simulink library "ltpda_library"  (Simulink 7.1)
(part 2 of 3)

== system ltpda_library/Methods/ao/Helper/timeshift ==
  In1 : Inport  OutDataType=sfix(16)  OutScaling=2^0
  timeshift : M-S-Function  Tag=timeshift  FunctionName=ltpdasim
  Out1 : Outport  OutDataType=sfix(16)  OutScaling=2^0
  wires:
  In1/1 -> timeshift/1
  timeshift/1 -> Out1/1

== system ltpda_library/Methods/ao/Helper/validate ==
  In1 : Inport  OutDataType=sfix(16)  OutScaling=2^0
  validate : M-S-Function  Tag=validate  FunctionName=ltpdasim
  Out1 : Outport  OutDataType=sfix(16)  OutScaling=2^0
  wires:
  In1/1 -> validate/1
  validate/1 -> Out1/1

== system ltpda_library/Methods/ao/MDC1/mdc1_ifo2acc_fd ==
  In1 : Inport  OutDataType=sfix(16)  OutScaling=2^0
  mdc1_ifo2acc_fd : M-S-Function  Tag=mdc1_ifo2acc_fd  FunctionName=ltpdasim
  Out1 : Outport  OutDataType=sfix(16)  OutScaling=2^0
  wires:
  In1/1 -> mdc1_ifo2acc_fd/1
  mdc1_ifo2acc_fd/1 -> Out1/1

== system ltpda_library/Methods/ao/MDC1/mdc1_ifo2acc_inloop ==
  In1 : Inport  OutDataType=sfix(16)  OutScaling=2^0
  mdc1_ifo2acc_inloop : M-S-Function  Tag=mdc1_ifo2acc_inloop  FunctionName=ltpdasim
  Out1 : Outport  OutDataType=sfix(16)  OutScaling=2^0
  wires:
  In1/1 -> mdc1_ifo2acc_inloop/1
  mdc1_ifo2acc_inloop/1 -> Out1/1

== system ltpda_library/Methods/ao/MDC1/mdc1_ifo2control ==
  In1 : Inport  OutDataType=sfix(16)  OutScaling=2^0
  mdc1_ifo2control : M-S-Function  Tag=mdc1_ifo2control  FunctionName=ltpdasim
  Out1 : Outport  OutDataType=sfix(16)  OutScaling=2^0
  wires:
  In1/1 -> mdc1_ifo2control/1
  mdc1_ifo2control/1 -> Out1/1

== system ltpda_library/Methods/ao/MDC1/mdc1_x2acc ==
  In1 : Inport  OutDataType=sfix(16)  OutScaling=2^0
  mdc1_x2acc : M-S-Function  Tag=mdc1_x2acc  FunctionName=ltpdasim
  Out1 : Outport  OutDataType=sfix(16)  OutScaling=2^0
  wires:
  In1/1 -> mdc1_x2acc/1
  mdc1_x2acc/1 -> Out1/1

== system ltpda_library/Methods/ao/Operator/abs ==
  In1 : Inport  OutDataType=sfix(16)  OutScaling=2^0
  abs : M-S-Function  Tag=abs  FunctionName=ltpdasim
  Out1 : Outport  OutDataType=sfix(16)  OutScaling=2^0
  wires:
  In1/1 -> abs/1
  abs/1 -> Out1/1

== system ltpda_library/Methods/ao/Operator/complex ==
  In1 : Inport  OutDataType=sfix(16)  OutScaling=2^0
  complex : M-S-Function  Tag=complex  FunctionName=ltpdasim
  Out1 : Outport  OutDataType=sfix(16)  OutScaling=2^0
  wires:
  In1/1 -> complex/1
  complex/1 -> Out1/1

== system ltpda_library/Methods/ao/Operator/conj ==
  In1 : Inport  OutDataType=sfix(16)  OutScaling=2^0
  conj : M-S-Function  Tag=conj  FunctionName=ltpdasim
  Out1 : Outport  OutDataType=sfix(16)  OutScaling=2^0
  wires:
  In1/1 -> conj/1
  conj/1 -> Out1/1

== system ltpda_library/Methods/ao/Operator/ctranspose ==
  In1 : Inport  OutDataType=sfix(16)  OutScaling=2^0
  ctranspose : M-S-Function  Tag=ctranspose  FunctionName=ltpdasim
  Out1 : Outport  OutDataType=sfix(16)  OutScaling=2^0
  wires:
  In1/1 -> ctranspose/1
  ctranspose/1 -> Out1/1

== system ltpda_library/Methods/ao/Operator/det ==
  In1 : Inport  OutDataType=sfix(16)  OutScaling=2^0
  det : M-S-Function  Tag=det  FunctionName=ltpdasim
  Out1 : Outport  OutDataType=sfix(16)  OutScaling=2^0
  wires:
  In1/1 -> det/1
  det/1 -> Out1/1

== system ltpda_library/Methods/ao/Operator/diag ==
  In1 : Inport  OutDataType=sfix(16)  OutScaling=2^0
  diag : M-S-Function  Tag=diag  FunctionName=ltpdasim
  Out1 : Outport  OutDataType=sfix(16)  OutScaling=2^0
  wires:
  In1/1 -> diag/1
  diag/1 -> Out1/1

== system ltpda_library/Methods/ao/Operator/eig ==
  In1 : Inport  OutDataType=sfix(16)  OutScaling=2^0
  eig : M-S-Function  Tag=eig  FunctionName=ltpdasim
  Out1 : Outport  OutDataType=sfix(16)  OutScaling=2^0
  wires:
  In1/1 -> eig/1
  eig/1 -> Out1/1

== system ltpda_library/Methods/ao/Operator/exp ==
  In1 : Inport  OutDataType=sfix(16)  OutScaling=2^0
  exp : M-S-Function  Tag=exp  FunctionName=ltpdasim
  Out1 : Outport  OutDataType=sfix(16)  OutScaling=2^0
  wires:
  In1/1 -> exp/1
  exp/1 -> Out1/1

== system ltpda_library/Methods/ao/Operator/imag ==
  In1 : Inport  OutDataType=sfix(16)  OutScaling=2^0
  imag : M-S-Function  Tag=imag  FunctionName=ltpdasim
  Out1 : Outport  OutDataType=sfix(16)  OutScaling=2^0
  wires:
  In1/1 -> imag/1
  imag/1 -> Out1/1

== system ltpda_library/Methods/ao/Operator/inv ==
  In1 : Inport  OutDataType=sfix(16)  OutScaling=2^0
  inv : M-S-Function  Tag=inv  FunctionName=ltpdasim
  Out1 : Outport  OutDataType=sfix(16)  OutScaling=2^0
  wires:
  In1/1 -> inv/1
  inv/1 -> Out1/1

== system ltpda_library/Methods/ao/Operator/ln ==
  In1 : Inport  OutDataType=sfix(16)  OutScaling=2^0
  ln : M-S-Function  Tag=ln  FunctionName=ltpdasim
  Out1 : Outport  OutDataType=sfix(16)  OutScaling=2^0
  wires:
  In1/1 -> ln/1
  ln/1 -> Out1/1

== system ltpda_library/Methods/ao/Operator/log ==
  In1 : Inport  OutDataType=sfix(16)  OutScaling=2^0
  log : M-S-Function  Tag=log  FunctionName=ltpdasim
  Out1 : Outport  OutDataType=sfix(16)  OutScaling=2^0
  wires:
  In1/1 -> log/1
  log/1 -> Out1/1

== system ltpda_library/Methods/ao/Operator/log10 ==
  In1 : Inport  OutDataType=sfix(16)  OutScaling=2^0
  log10 : M-S-Function  Tag=log10  FunctionName=ltpdasim
  Out1 : Outport  OutDataType=sfix(16)  OutScaling=2^0
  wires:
  In1/1 -> log10/1
  log10/1 -> Out1/1

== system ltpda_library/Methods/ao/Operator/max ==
  In1 : Inport  OutDataType=sfix(16)  OutScaling=2^0
  max : M-S-Function  Tag=max  FunctionName=ltpdasim
  Out1 : Outport  OutDataType=sfix(16)  OutScaling=2^0
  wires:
  In1/1 -> max/1
  max/1 -> Out1/1

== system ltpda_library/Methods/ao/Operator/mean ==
  In1 : Inport  OutDataType=sfix(16)  OutScaling=2^0
  mean : M-S-Function  Tag=mean  FunctionName=ltpdasim
  Out1 : Outport  OutDataType=sfix(16)  OutScaling=2^0
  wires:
  In1/1 -> mean/1
  mean/1 -> Out1/1

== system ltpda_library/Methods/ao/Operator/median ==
  In1 : Inport  OutDataType=sfix(16)  OutScaling=2^0
  median : M-S-Function  Tag=median  FunctionName=ltpdasim
  Out1 : Outport  OutDataType=sfix(16)  OutScaling=2^0
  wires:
  In1/1 -> median/1
  median/1 -> Out1/1

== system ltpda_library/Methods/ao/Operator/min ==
  In1 : Inport  OutDataType=sfix(16)  OutScaling=2^0
  min : M-S-Function  Tag=min  FunctionName=ltpdasim
  Out1 : Outport  OutDataType=sfix(16)  OutScaling=2^0
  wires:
  In1/1 -> min/1
  min/1 -> Out1/1

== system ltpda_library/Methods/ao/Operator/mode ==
  In1 : Inport  OutDataType=sfix(16)  OutScaling=2^0
  mode : M-S-Function  Tag=mode  FunctionName=ltpdasim
  Out1 : Outport  OutDataType=sfix(16)  OutScaling=2^0
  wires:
  In1/1 -> mode/1
  mode/1 -> Out1/1

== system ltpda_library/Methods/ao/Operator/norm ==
  In1 : Inport  OutDataType=sfix(16)  OutScaling=2^0
  norm : M-S-Function  Tag=norm  FunctionName=ltpdasim
  Out1 : Outport  OutDataType=sfix(16)  OutScaling=2^0
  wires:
  In1/1 -> norm/1
  norm/1 -> Out1/1

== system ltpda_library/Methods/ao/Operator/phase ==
  In1 : Inport  OutDataType=sfix(16)  OutScaling=2^0
  phase : M-S-Function  Tag=phase  FunctionName=ltpdasim
  Out1 : Outport  OutDataType=sfix(16)  OutScaling=2^0
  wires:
  In1/1 -> phase/1
  phase/1 -> Out1/1

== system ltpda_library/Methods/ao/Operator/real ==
  In1 : Inport  OutDataType=sfix(16)  OutScaling=2^0
  real : M-S-Function  Tag=real  FunctionName=ltpdasim
  Out1 : Outport  OutDataType=sfix(16)  OutScaling=2^0
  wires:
  In1/1 -> real/1
  real/1 -> Out1/1

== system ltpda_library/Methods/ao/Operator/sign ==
  In1 : Inport  OutDataType=sfix(16)  OutScaling=2^0
  sign : M-S-Function  Tag=sign  FunctionName=ltpdasim
  Out1 : Outport  OutDataType=sfix(16)  OutScaling=2^0
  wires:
  In1/1 -> sign/1
  sign/1 -> Out1/1

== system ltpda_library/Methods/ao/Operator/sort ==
  In1 : Inport  OutDataType=sfix(16)  OutScaling=2^0
  sort : M-S-Function  Tag=sort  FunctionName=ltpdasim
  Out1 : Outport  OutDataType=sfix(16)  OutScaling=2^0
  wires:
  In1/1 -> sort/1
  sort/1 -> Out1/1

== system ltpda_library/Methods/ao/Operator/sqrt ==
  In1 : Inport  OutDataType=sfix(16)  OutScaling=2^0
  sqrt : M-S-Function  Tag=sqrt  FunctionName=ltpdasim
  Out1 : Outport  OutDataType=sfix(16)  OutScaling=2^0
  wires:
  In1/1 -> sqrt/1
  sqrt/1 -> Out1/1

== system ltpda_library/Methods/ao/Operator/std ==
  In1 : Inport  OutDataType=sfix(16)  OutScaling=2^0
  std : M-S-Function  Tag=std  FunctionName=ltpdasim
  Out1 : Outport  OutDataType=sfix(16)  OutScaling=2^0
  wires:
  In1/1 -> std/1
  std/1 -> Out1/1

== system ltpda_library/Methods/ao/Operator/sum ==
  In1 : Inport  OutDataType=sfix(16)  OutScaling=2^0
  sum : M-S-Function  Tag=sum  FunctionName=ltpdasim
  Out1 : Outport  OutDataType=sfix(16)  OutScaling=2^0
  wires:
  In1/1 -> sum/1
  sum/1 -> Out1/1

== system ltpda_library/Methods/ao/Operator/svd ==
  In1 : Inport  OutDataType=sfix(16)  OutScaling=2^0
  svd : M-S-Function  Tag=svd  FunctionName=ltpdasim
  Out1 : Outport  OutDataType=sfix(16)  OutScaling=2^0
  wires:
  In1/1 -> svd/1
  svd/1 -> Out1/1

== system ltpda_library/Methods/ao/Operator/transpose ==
  In1 : Inport  OutDataType=sfix(16)  OutScaling=2^0
  transpose : M-S-Function  Tag=transpose  FunctionName=ltpdasim
  Out1 : Outport  OutDataType=sfix(16)  OutScaling=2^0
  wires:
  In1/1 -> transpose/1
  transpose/1 -> Out1/1

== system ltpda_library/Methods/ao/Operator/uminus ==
  In1 : Inport  OutDataType=sfix(16)  OutScaling=2^0
  uminus : M-S-Function  Tag=uminus  FunctionName=ltpdasim
  Out1 : Outport  OutDataType=sfix(16)  OutScaling=2^0
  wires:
  In1/1 -> uminus/1
  uminus/1 -> Out1/1

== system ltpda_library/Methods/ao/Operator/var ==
  In1 : Inport  OutDataType=sfix(16)  OutScaling=2^0
  var : M-S-Function  Tag=var  FunctionName=ltpdasim
  Out1 : Outport  OutDataType=sfix(16)  OutScaling=2^0
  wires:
  In1/1 -> var/1
  var/1 -> Out1/1

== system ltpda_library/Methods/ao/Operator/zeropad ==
  In1 : Inport  OutDataType=sfix(16)  OutScaling=2^0
  zeropad : M-S-Function  Tag=zeropad  FunctionName=ltpdasim
  Out1 : Outport  OutDataType=sfix(16)  OutScaling=2^0
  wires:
  In1/1 -> zeropad/1
  zeropad/1 -> Out1/1

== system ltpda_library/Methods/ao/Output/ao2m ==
  In1 : Inport  OutDataType=sfix(16)  OutScaling=2^0
  Terminator : Terminator
  ao2m : M-S-Function  Tag=ao2m  FunctionName=ltpdasim
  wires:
  ao2m/1 -> Terminator/1
  In1/1 -> ao2m/1

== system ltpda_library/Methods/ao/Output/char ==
  In1 : Inport  OutDataType=sfix(16)  OutScaling=2^0
  Terminator : Terminator
  char : M-S-Function  Tag=char  FunctionName=ltpdasim
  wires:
  char/1 -> Terminator/1
  In1/1 -> char/1

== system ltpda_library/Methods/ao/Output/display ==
  In1 : Inport  OutDataType=sfix(16)  OutScaling=2^0
  Terminator : Terminator
  display : M-S-Function  Tag=display  FunctionName=ltpdasim
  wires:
  display/1 -> Terminator/1
  In1/1 -> display/1

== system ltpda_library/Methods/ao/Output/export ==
  In1 : Inport  OutDataType=sfix(16)  OutScaling=2^0
  Terminator : Terminator
  export : M-S-Function  Tag=export  FunctionName=ltpdasim
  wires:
  export/1 -> Terminator/1
  In1/1 -> export/1

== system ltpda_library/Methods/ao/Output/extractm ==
  In1 : Inport  OutDataType=sfix(16)  OutScaling=2^0
  Terminator : Terminator
  extractm : M-S-Function  Tag=extractm  FunctionName=ltpdasim
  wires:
  extractm/1 -> Terminator/1
  In1/1 -> extractm/1

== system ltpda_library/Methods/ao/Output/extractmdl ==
  In1 : Inport  OutDataType=sfix(16)  OutScaling=2^0
  Terminator : Terminator
  extractmdl : M-S-Function  Tag=extractmdl  FunctionName=ltpdasim
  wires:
  extractmdl/1 -> Terminator/1
  In1/1 -> extractmdl/1

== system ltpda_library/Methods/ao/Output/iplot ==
  In1 : Inport  OutDataType=sfix(16)  OutScaling=2^0
  Terminator : Terminator
  iplot : M-S-Function  Tag=iplot  FunctionName=ltpdasim
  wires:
  iplot/1 -> Terminator/1
  In1/1 -> iplot/1

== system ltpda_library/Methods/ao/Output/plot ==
  In1 : Inport  OutDataType=sfix(16)  OutScaling=2^0
  Terminator : Terminator
  plot : M-S-Function  Tag=plot  FunctionName=ltpdasim
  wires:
  plot/1 -> Terminator/1
  In1/1 -> plot/1

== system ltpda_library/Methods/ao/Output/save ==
  In1 : Inport  OutDataType=sfix(16)  OutScaling=2^0
  Terminator : Terminator
  save : M-S-Function  Tag=save  FunctionName=ltpdasim
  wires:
  save/1 -> Terminator/1
  In1/1 -> save/1

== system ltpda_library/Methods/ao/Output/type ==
  In1 : Inport  OutDataType=sfix(16)  OutScaling=2^0
  Terminator : Terminator
  type : M-S-Function  Tag=type  FunctionName=ltpdasim
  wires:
  type/1 -> Terminator/1
  In1/1 -> type/1

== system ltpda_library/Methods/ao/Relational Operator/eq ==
  In1 : Inport  OutDataType=sfix(16)  OutScaling=2^0
  eq : M-S-Function  Tag=eq  FunctionName=ltpdasim
  Out1 : Outport  OutDataType=sfix(16)  OutScaling=2^0
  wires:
  In1/1 -> eq/1
  eq/1 -> Out1/1

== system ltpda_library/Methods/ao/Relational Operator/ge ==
  In1 : Inport  OutDataType=sfix(16)  OutScaling=2^0
  ge : M-S-Function  Tag=ge  FunctionName=ltpdasim
  Out1 : Outport  OutDataType=sfix(16)  OutScaling=2^0
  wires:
  In1/1 -> ge/1
  ge/1 -> Out1/1

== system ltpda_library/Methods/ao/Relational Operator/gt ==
  In1 : Inport  OutDataType=sfix(16)  OutScaling=2^0
  gt : M-S-Function  Tag=gt  FunctionName=ltpdasim
  Out1 : Outport  OutDataType=sfix(16)  OutScaling=2^0
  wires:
  In1/1 -> gt/1
  gt/1 -> Out1/1

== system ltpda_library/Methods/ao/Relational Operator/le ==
  In1 : Inport  OutDataType=sfix(16)  OutScaling=2^0
  le : M-S-Function  Tag=le  FunctionName=ltpdasim
  Out1 : Outport  OutDataType=sfix(16)  OutScaling=2^0
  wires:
  In1/1 -> le/1
  le/1 -> Out1/1

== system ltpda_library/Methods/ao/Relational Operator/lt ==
  In1 : Inport  OutDataType=sfix(16)  OutScaling=2^0
  lt : M-S-Function  Tag=lt  FunctionName=ltpdasim
  Out1 : Outport  OutDataType=sfix(16)  OutScaling=2^0
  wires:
  In1/1 -> lt/1
  lt/1 -> Out1/1

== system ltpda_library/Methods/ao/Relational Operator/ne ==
  In1 : Inport  OutDataType=sfix(16)  OutScaling=2^0
  ne : M-S-Function  Tag=ne  FunctionName=ltpdasim
  Out1 : Outport  OutDataType=sfix(16)  OutScaling=2^0
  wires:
  In1/1 -> ne/1
  ne/1 -> Out1/1

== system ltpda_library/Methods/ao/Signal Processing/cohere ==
  In1 : Inport  OutDataType=sfix(16)  OutScaling=2^0
  cohere : M-S-Function  Tag=cohere  FunctionName=ltpdasim
  Out1 : Outport  OutDataType=sfix(16)  OutScaling=2^0
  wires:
  In1/1 -> cohere/1
  cohere/1 -> Out1/1

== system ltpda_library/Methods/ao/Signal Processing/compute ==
  In1 : Inport  OutDataType=sfix(16)  OutScaling=2^0
  compute : M-S-Function  Tag=compute  FunctionName=ltpdasim
  Out1 : Outport  OutDataType=sfix(16)  OutScaling=2^0
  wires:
  In1/1 -> compute/1
  compute/1 -> Out1/1

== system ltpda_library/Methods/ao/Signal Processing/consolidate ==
  In1 : Inport  OutDataType=sfix(16)  OutScaling=2^0
  consolidate : M-S-Function  Tag=consolidate  FunctionName=ltpdasim
  Out1 : Outport  OutDataType=sfix(16)  OutScaling=2^0
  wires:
  In1/1 -> consolidate/1
  consolidate/1 -> Out1/1

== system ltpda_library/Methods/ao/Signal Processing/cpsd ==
  In1 : Inport  OutDataType=sfix(16)  OutScaling=2^0
  cpsd : M-S-Function  Tag=cpsd  FunctionName=ltpdasim
  Out1 : Outport  OutDataType=sfix(16)  OutScaling=2^0
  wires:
  In1/1 -> cpsd/1
  cpsd/1 -> Out1/1

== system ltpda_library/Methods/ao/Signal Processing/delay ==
  In1 : Inport  OutDataType=sfix(16)  OutScaling=2^0
  delay : M-S-Function  Tag=delay  FunctionName=ltpdasim
  Out1 : Outport  OutDataType=sfix(16)  OutScaling=2^0
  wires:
  In1/1 -> delay/1
  delay/1 -> Out1/1

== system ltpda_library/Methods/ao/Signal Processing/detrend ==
  In1 : Inport  OutDataType=sfix(16)  OutScaling=2^0
  detrend : M-S-Function  Tag=detrend  FunctionName=ltpdasim
  Out1 : Outport  OutDataType=sfix(16)  OutScaling=2^0
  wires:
  In1/1 -> detrend/1
  detrend/1 -> Out1/1

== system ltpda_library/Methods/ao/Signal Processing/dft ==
  In1 : Inport  OutDataType=sfix(16)  OutScaling=2^0
  dft : M-S-Function  Tag=dft  FunctionName=ltpdasim
  Out1 : Outport  OutDataType=sfix(16)  OutScaling=2^0
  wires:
  In1/1 -> dft/1
  dft/1 -> Out1/1

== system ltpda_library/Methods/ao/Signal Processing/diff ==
  In1 : Inport  OutDataType=sfix(16)  OutScaling=2^0
  diff : M-S-Function  Tag=diff  FunctionName=ltpdasim
  Out1 : Outport  OutDataType=sfix(16)  OutScaling=2^0
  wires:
  In1/1 -> diff/1
  diff/1 -> Out1/1

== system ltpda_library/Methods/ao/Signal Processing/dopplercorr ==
  In1 : Inport  OutDataType=sfix(16)  OutScaling=2^0
  dopplercorr : M-S-Function  Tag=dopplercorr  FunctionName=ltpdasim
  Out1 : Outport  OutDataType=sfix(16)  OutScaling=2^0
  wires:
  In1/1 -> dopplercorr/1
  dopplercorr/1 -> Out1/1

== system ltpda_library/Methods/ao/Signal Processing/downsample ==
  In1 : Inport  OutDataType=sfix(16)  OutScaling=2^0
  downsample : M-S-Function  Tag=downsample  FunctionName=ltpdasim
  Out1 : Outport  OutDataType=sfix(16)  OutScaling=2^0
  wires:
  In1/1 -> downsample/1
  downsample/1 -> Out1/1

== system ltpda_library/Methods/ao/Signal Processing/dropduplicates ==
  In1 : Inport  OutDataType=sfix(16)  OutScaling=2^0
  dropduplicates : M-S-Function  Tag=dropduplicates  FunctionName=ltpdasim
  Out1 : Outport  OutDataType=sfix(16)  OutScaling=2^0
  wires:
  In1/1 -> dropduplicates/1
  dropduplicates/1 -> Out1/1

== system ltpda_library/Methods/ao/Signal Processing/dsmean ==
  In1 : Inport  OutDataType=sfix(16)  OutScaling=2^0
  dsmean : M-S-Function  Tag=dsmean  FunctionName=ltpdasim
  Out1 : Outport  OutDataType=sfix(16)  OutScaling=2^0
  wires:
  In1/1 -> dsmean/1
  dsmean/1 -> Out1/1

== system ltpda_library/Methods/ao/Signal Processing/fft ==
  In1 : Inport  OutDataType=sfix(16)  OutScaling=2^0
  fft : M-S-Function  Tag=fft  FunctionName=ltpdasim
  Out1 : Outport  OutDataType=sfix(16)  OutScaling=2^0
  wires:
  In1/1 -> fft/1
  fft/1 -> Out1/1

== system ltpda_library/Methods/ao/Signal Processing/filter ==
  In1 : Inport  OutDataType=sfix(16)  OutScaling=2^0
  filter : M-S-Function  Tag=filter  FunctionName=ltpdasim
  Out1 : Outport  OutDataType=sfix(16)  OutScaling=2^0
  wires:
  In1/1 -> filter/1
  filter/1 -> Out1/1

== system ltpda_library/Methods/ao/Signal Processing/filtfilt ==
  In1 : Inport  OutDataType=sfix(16)  OutScaling=2^0
  filtfilt : M-S-Function  Tag=filtfilt  FunctionName=ltpdasim
  Out1 : Outport  OutDataType=sfix(16)  OutScaling=2^0
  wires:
  In1/1 -> filtfilt/1
  filtfilt/1 -> Out1/1

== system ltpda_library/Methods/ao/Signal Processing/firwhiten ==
  In1 : Inport  OutDataType=sfix(16)  OutScaling=2^0
  firwhiten : M-S-Function  Tag=firwhiten  FunctionName=ltpdasim
  Out1 : Outport  OutDataType=sfix(16)  OutScaling=2^0
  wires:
  In1/1 -> firwhiten/1
  firwhiten/1 -> Out1/1

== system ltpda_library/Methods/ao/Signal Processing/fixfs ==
  In1 : Inport  OutDataType=sfix(16)  OutScaling=2^0
  fixfs : M-S-Function  Tag=fixfs  FunctionName=ltpdasim
  Out1 : Outport  OutDataType=sfix(16)  OutScaling=2^0
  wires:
  In1/1 -> fixfs/1
  fixfs/1 -> Out1/1

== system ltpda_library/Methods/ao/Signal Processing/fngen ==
  In1 : Inport  OutDataType=sfix(16)  OutScaling=2^0
  fngen : M-S-Function  Tag=fngen  FunctionName=ltpdasim
  Out1 : Outport  OutDataType=sfix(16)  OutScaling=2^0
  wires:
  In1/1 -> fngen/1
  fngen/1 -> Out1/1

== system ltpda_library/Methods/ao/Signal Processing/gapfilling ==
  In1 : Inport  OutDataType=sfix(16)  OutScaling=2^0
  gapfilling : M-S-Function  Tag=gapfilling  FunctionName=ltpdasim
  Out1 : Outport  OutDataType=sfix(16)  OutScaling=2^0
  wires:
  In1/1 -> gapfilling/1
  gapfilling/1 -> Out1/1

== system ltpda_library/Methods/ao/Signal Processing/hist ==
  In1 : Inport  OutDataType=sfix(16)  OutScaling=2^0
  hist : M-S-Function  Tag=hist  FunctionName=ltpdasim
  Out1 : Outport  OutDataType=sfix(16)  OutScaling=2^0
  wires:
  In1/1 -> hist/1
  hist/1 -> Out1/1

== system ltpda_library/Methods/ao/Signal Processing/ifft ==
  In1 : Inport  OutDataType=sfix(16)  OutScaling=2^0
  ifft : M-S-Function  Tag=ifft  FunctionName=ltpdasim
  Out1 : Outport  OutDataType=sfix(16)  OutScaling=2^0
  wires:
  In1/1 -> ifft/1
  ifft/1 -> Out1/1

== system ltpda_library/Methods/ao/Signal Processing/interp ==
  In1 : Inport  OutDataType=sfix(16)  OutScaling=2^0
  interp : M-S-Function  Tag=interp  FunctionName=ltpdasim
  Out1 : Outport  OutDataType=sfix(16)  OutScaling=2^0
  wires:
  In1/1 -> interp/1
  interp/1 -> Out1/1

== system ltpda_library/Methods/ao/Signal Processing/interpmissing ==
  In1 : Inport  OutDataType=sfix(16)  OutScaling=2^0
  interpmissing : M-S-Function  Tag=interpmissing  FunctionName=ltpdasim
  Out1 : Outport  OutDataType=sfix(16)  OutScaling=2^0
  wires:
  In1/1 -> interpmissing/1
  interpmissing/1 -> Out1/1

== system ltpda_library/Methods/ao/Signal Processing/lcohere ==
  In1 : Inport  OutDataType=sfix(16)  OutScaling=2^0
  lcohere : M-S-Function  Tag=lcohere  FunctionName=ltpdasim
  Out1 : Outport  OutDataType=sfix(16)  OutScaling=2^0
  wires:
  In1/1 -> lcohere/1
  lcohere/1 -> Out1/1

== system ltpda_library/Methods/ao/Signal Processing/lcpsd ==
  In1 : Inport  OutDataType=sfix(16)  OutScaling=2^0
  lcpsd : M-S-Function  Tag=lcpsd  FunctionName=ltpdasim
  Out1 : Outport  OutDataType=sfix(16)  OutScaling=2^0
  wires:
  In1/1 -> lcpsd/1
  lcpsd/1 -> Out1/1

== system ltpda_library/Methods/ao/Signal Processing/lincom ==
  In1 : Inport  OutDataType=sfix(16)  OutScaling=2^0
  lincom : M-S-Function  Tag=lincom  FunctionName=ltpdasim
  Out1 : Outport  OutDataType=sfix(16)  OutScaling=2^0
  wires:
  In1/1 -> lincom/1
  lincom/1 -> Out1/1

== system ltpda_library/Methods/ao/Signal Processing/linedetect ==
  In1 : Inport  OutDataType=sfix(16)  OutScaling=2^0
  linedetect : M-S-Function  Tag=linedetect  FunctionName=ltpdasim
  Out1 : Outport  OutDataType=sfix(16)  OutScaling=2^0
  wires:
  In1/1 -> linedetect/1
  linedetect/1 -> Out1/1

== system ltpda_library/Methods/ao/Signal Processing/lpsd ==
  In1 : Inport  OutDataType=sfix(16)  OutScaling=2^0
  lpsd : M-S-Function  Tag=lpsd  FunctionName=ltpdasim
  Out1 : Outport  OutDataType=sfix(16)  OutScaling=2^0
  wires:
  In1/1 -> lpsd/1
  lpsd/1 -> Out1/1

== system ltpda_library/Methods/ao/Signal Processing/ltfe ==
  In1 : Inport  OutDataType=sfix(16)  OutScaling=2^0
  ltfe : M-S-Function  Tag=ltfe  FunctionName=ltpdasim
  Out1 : Outport  OutDataType=sfix(16)  OutScaling=2^0
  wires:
  In1/1 -> ltfe/1
  ltfe/1 -> Out1/1

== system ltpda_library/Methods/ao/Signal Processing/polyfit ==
  In1 : Inport  OutDataType=sfix(16)  OutScaling=2^0
  polyfit : M-S-Function  Tag=polyfit  FunctionName=ltpdasim
  Out1 : Outport  OutDataType=sfix(16)  OutScaling=2^0
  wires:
  In1/1 -> polyfit/1
  polyfit/1 -> Out1/1

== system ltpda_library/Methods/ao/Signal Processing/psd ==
  In1 : Inport  OutDataType=sfix(16)  OutScaling=2^0
  psd : M-S-Function  Tag=psd  FunctionName=ltpdasim
  Out1 : Outport  OutDataType=sfix(16)  OutScaling=2^0
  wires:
  In1/1 -> psd/1
  psd/1 -> Out1/1

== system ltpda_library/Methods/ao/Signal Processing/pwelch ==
  In1 : Inport  OutDataType=sfix(16)  OutScaling=2^0
  pwelch : M-S-Function  Tag=pwelch  FunctionName=ltpdasim
  Out1 : Outport  OutDataType=sfix(16)  OutScaling=2^0
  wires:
  In1/1 -> pwelch/1
  pwelch/1 -> Out1/1

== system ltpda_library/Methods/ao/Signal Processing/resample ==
  In1 : Inport  OutDataType=sfix(16)  OutScaling=2^0
  resample : M-S-Function  Tag=resample  FunctionName=ltpdasim
  Out1 : Outport  OutDataType=sfix(16)  OutScaling=2^0
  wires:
  In1/1 -> resample/1
  resample/1 -> Out1/1

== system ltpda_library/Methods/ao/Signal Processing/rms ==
  In1 : Inport  OutDataType=sfix(16)  OutScaling=2^0
  rms : M-S-Function  Tag=rms  FunctionName=ltpdasim
  Out1 : Outport  OutDataType=sfix(16)  OutScaling=2^0
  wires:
  In1/1 -> rms/1
  rms/1 -> Out1/1

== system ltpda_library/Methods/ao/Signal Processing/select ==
  In1 : Inport  OutDataType=sfix(16)  OutScaling=2^0
  select : M-S-Function  Tag=select  FunctionName=ltpdasim
  Out1 : Outport  OutDataType=sfix(16)  OutScaling=2^0
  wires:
  In1/1 -> select/1
  select/1 -> Out1/1

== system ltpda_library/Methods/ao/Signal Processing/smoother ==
  In1 : Inport  OutDataType=sfix(16)  OutScaling=2^0
  smoother : M-S-Function  Tag=smoother  FunctionName=ltpdasim
  Out1 : Outport  OutDataType=sfix(16)  OutScaling=2^0
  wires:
  In1/1 -> smoother/1
  smoother/1 -> Out1/1

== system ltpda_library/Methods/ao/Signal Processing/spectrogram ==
  In1 : Inport  OutDataType=sfix(16)  OutScaling=2^0
  spectrogram : M-S-Function  Tag=spectrogram  FunctionName=ltpdasim
  Out1 : Outport  OutDataType=sfix(16)  OutScaling=2^0
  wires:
  In1/1 -> spectrogram/1
  spectrogram/1 -> Out1/1

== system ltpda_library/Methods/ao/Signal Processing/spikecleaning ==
  In1 : Inport  OutDataType=sfix(16)  OutScaling=2^0
  spikecleaning : M-S-Function  Tag=spikecleaning  FunctionName=ltpdasim
  Out1 : Outport  OutDataType=sfix(16)  OutScaling=2^0
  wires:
  In1/1 -> spikecleaning/1
  spikecleaning/1 -> Out1/1

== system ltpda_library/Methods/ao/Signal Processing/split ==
  In1 : Inport  OutDataType=sfix(16)  OutScaling=2^0
  split : M-S-Function  Tag=split  FunctionName=ltpdasim
  Out1 : Outport  OutDataType=sfix(16)  OutScaling=2^0
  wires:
  In1/1 -> split/1
  split/1 -> Out1/1

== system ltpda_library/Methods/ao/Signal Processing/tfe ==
  In1 : Inport  OutDataType=sfix(16)  OutScaling=2^0
  tfe : M-S-Function  Tag=tfe  FunctionName=ltpdasim
  Out1 : Outport  OutDataType=sfix(16)  OutScaling=2^0
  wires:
  In1/1 -> tfe/1
  tfe/1 -> Out1/1

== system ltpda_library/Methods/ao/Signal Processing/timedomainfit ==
  In1 : Inport  OutDataType=sfix(16)  OutScaling=2^0
  timedomainfit : M-S-Function  Tag=timedomainfit  FunctionName=ltpdasim
  Out1 : Outport  OutDataType=sfix(16)  OutScaling=2^0
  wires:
  In1/1 -> timedomainfit/1
  timedomainfit/1 -> Out1/1

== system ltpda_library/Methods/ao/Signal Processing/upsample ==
  In1 : Inport  OutDataType=sfix(16)  OutScaling=2^0
  upsample : M-S-Function  Tag=upsample  FunctionName=ltpdasim
  Out1 : Outport  OutDataType=sfix(16)  OutScaling=2^0
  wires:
  In1/1 -> upsample/1
  upsample/1 -> Out1/1

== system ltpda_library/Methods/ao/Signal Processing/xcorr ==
  In1 : Inport  OutDataType=sfix(16)  OutScaling=2^0
  xcorr : M-S-Function  Tag=xcorr  FunctionName=ltpdasim
  Out1 : Outport  OutDataType=sfix(16)  OutScaling=2^0
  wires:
  In1/1 -> xcorr/1
  xcorr/1 -> Out1/1

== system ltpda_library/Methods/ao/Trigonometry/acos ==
  In1 : Inport  OutDataType=sfix(16)  OutScaling=2^0
  acos : M-S-Function  Tag=acos  FunctionName=ltpdasim
  Out1 : Outport  OutDataType=sfix(16)  OutScaling=2^0
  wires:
  In1/1 -> acos/1
  acos/1 -> Out1/1

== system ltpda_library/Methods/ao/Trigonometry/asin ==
  In1 : Inport  OutDataType=sfix(16)  OutScaling=2^0
  asin : M-S-Function  Tag=asin  FunctionName=ltpdasim
  Out1 : Outport  OutDataType=sfix(16)  OutScaling=2^0
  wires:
  In1/1 -> asin/1
  asin/1 -> Out1/1

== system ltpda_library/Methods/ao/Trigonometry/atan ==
  In1 : Inport  OutDataType=sfix(16)  OutScaling=2^0
  atan : M-S-Function  Tag=atan  FunctionName=ltpdasim
  Out1 : Outport  OutDataType=sfix(16)  OutScaling=2^0
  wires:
  In1/1 -> atan/1
  atan/1 -> Out1/1

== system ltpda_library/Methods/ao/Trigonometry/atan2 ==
  In1 : Inport  OutDataType=sfix(16)  OutScaling=2^0
  atan2 : M-S-Function  Tag=atan2  FunctionName=ltpdasim
  Out1 : Outport  OutDataType=sfix(16)  OutScaling=2^0
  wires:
  In1/1 -> atan2/1
  atan2/1 -> Out1/1

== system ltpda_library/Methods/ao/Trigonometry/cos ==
  In1 : Inport  OutDataType=sfix(16)  OutScaling=2^0
  cos : M-S-Function  Tag=cos  FunctionName=ltpdasim
  Out1 : Outport  OutDataType=sfix(16)  OutScaling=2^0
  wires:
  In1/1 -> cos/1
  cos/1 -> Out1/1

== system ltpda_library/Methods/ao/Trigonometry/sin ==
  In1 : Inport  OutDataType=sfix(16)  OutScaling=2^0
  sin : M-S-Function  Tag=sin  FunctionName=ltpdasim
  Out1 : Outport  OutDataType=sfix(16)  OutScaling=2^0
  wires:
  In1/1 -> sin/1
  sin/1 -> Out1/1

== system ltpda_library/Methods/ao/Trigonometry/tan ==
  In1 : Inport  OutDataType=sfix(16)  OutScaling=2^0
  tan : M-S-Function  Tag=tan  FunctionName=ltpdasim
  Out1 : Outport  OutDataType=sfix(16)  OutScaling=2^0
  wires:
  In1/1 -> tan/1
  tan/1 -> Out1/1

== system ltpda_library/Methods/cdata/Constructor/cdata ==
  Ground : Ground
  cdata : M-S-Function  Tag=cdata  FunctionName=ltpdasim
  Out1 : Outport  OutDataType=sfix(16)  OutScaling=2^0
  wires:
  Ground/1 -> cdata/1
  cdata/1 -> Out1/1

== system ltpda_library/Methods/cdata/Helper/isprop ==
  In1 : Inport  OutDataType=sfix(16)  OutScaling=2^0
  isprop : M-S-Function  Tag=isprop  FunctionName=ltpdasim
  Out1 : Outport  OutDataType=sfix(16)  OutScaling=2^0
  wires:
  In1/1 -> isprop/1
  isprop/1 -> Out1/1

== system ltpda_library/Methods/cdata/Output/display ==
  In1 : Inport  OutDataType=sfix(16)  OutScaling=2^0
  Terminator : Terminator
  display : M-S-Function  Tag=display  FunctionName=ltpdasim
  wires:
  display/1 -> Terminator/1
  In1/1 -> display/1

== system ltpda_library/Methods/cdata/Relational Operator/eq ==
  In1 : Inport  OutDataType=sfix(16)  OutScaling=2^0
  eq : M-S-Function  Tag=eq  FunctionName=ltpdasim
  Out1 : Outport  OutDataType=sfix(16)  OutScaling=2^0
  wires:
  In1/1 -> eq/1
  eq/1 -> Out1/1

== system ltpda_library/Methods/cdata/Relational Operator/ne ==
  In1 : Inport  OutDataType=sfix(16)  OutScaling=2^0
  ne : M-S-Function  Tag=ne  FunctionName=ltpdasim
  Out1 : Outport  OutDataType=sfix(16)  OutScaling=2^0
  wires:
  In1/1 -> ne/1
  ne/1 -> Out1/1

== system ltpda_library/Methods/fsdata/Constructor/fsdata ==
  Ground : Ground
  fsdata : M-S-Function  Tag=fsdata  FunctionName=ltpdasim
  Out1 : Outport  OutDataType=sfix(16)  OutScaling=2^0
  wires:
  Ground/1 -> fsdata/1
  fsdata/1 -> Out1/1

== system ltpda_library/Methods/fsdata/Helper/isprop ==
  In1 : Inport  OutDataType=sfix(16)  OutScaling=2^0
  isprop : M-S-Function  Tag=isprop  FunctionName=ltpdasim
  Out1 : Outport  OutDataType=sfix(16)  OutScaling=2^0
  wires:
  In1/1 -> isprop/1
  isprop/1 -> Out1/1

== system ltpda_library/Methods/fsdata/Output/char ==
  In1 : Inport  OutDataType=sfix(16)  OutScaling=2^0
  Terminator : Terminator
  char : M-S-Function  Tag=char  FunctionName=ltpdasim
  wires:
  char/1 -> Terminator/1
  In1/1 -> char/1

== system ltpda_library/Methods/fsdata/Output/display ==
  In1 : Inport  OutDataType=sfix(16)  OutScaling=2^0
  Terminator : Terminator
  display : M-S-Function  Tag=display  FunctionName=ltpdasim
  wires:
  display/1 -> Terminator/1
  In1/1 -> display/1

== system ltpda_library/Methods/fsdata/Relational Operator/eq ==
  In1 : Inport  OutDataType=sfix(16)  OutScaling=2^0
  eq : M-S-Function  Tag=eq  FunctionName=ltpdasim
  Out1 : Outport  OutDataType=sfix(16)  OutScaling=2^0
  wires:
  In1/1 -> eq/1
  eq/1 -> Out1/1

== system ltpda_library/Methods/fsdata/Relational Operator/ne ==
  In1 : Inport  OutDataType=sfix(16)  OutScaling=2^0
  ne : M-S-Function  Tag=ne  FunctionName=ltpdasim
  Out1 : Outport  OutDataType=sfix(16)  OutScaling=2^0
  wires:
  In1/1 -> ne/1
  ne/1 -> Out1/1

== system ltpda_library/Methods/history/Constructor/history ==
  Ground : Ground
  history : M-S-Function  Tag=history  FunctionName=ltpdasim
  Out1 : Outport  OutDataType=sfix(16)  OutScaling=2^0
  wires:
  Ground/1 -> history/1
  history/1 -> Out1/1

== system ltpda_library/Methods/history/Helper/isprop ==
  In1 : Inport  OutDataType=sfix(16)  OutScaling=2^0
  isprop : M-S-Function  Tag=isprop  FunctionName=ltpdasim
  Out1 : Outport  OutDataType=sfix(16)  OutScaling=2^0
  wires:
  In1/1 -> isprop/1
  isprop/1 -> Out1/1

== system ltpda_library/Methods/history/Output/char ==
  In1 : Inport  OutDataType=sfix(16)  OutScaling=2^0
  Terminator : Terminator
  char : M-S-Function  Tag=char  FunctionName=ltpdasim
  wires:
  char/1 -> Terminator/1
  In1/1 -> char/1

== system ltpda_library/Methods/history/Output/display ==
  In1 : Inport  OutDataType=sfix(16)  OutScaling=2^0
  Terminator : Terminator
  display : M-S-Function  Tag=display  FunctionName=ltpdasim
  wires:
  display/1 -> Terminator/1
  In1/1 -> display/1

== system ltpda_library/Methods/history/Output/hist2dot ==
  In1 : Inport  OutDataType=sfix(16)  OutScaling=2^0
  Terminator : Terminator
  hist2dot : M-S-Function  Tag=hist2dot  FunctionName=ltpdasim
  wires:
  hist2dot/1 -> Terminator/1
  In1/1 -> hist2dot/1

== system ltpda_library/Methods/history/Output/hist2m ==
  In1 : Inport  OutDataType=sfix(16)  OutScaling=2^0
  Terminator : Terminator
  hist2m : M-S-Function  Tag=hist2m  FunctionName=ltpdasim
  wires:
  hist2m/1 -> Terminator/1
  In1/1 -> hist2m/1

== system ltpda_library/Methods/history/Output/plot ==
  In1 : Inport  OutDataType=sfix(16)  OutScaling=2^0
  Terminator : Terminator
  plot : M-S-Function  Tag=plot  FunctionName=ltpdasim
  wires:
  plot/1 -> Terminator/1
  In1/1 -> plot/1

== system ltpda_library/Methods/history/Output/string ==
  In1 : Inport  OutDataType=sfix(16)  OutScaling=2^0
  Terminator : Terminator
  string : M-S-Function  Tag=string  FunctionName=ltpdasim
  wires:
  string/1 -> Terminator/1
  In1/1 -> string/1

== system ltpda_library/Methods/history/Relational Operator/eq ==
  In1 : Inport  OutDataType=sfix(16)  OutScaling=2^0
  eq : M-S-Function  Tag=eq  FunctionName=ltpdasim
  Out1 : Outport  OutDataType=sfix(16)  OutScaling=2^0
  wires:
  In1/1 -> eq/1
  eq/1 -> Out1/1

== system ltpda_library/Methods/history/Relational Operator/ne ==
  In1 : Inport  OutDataType=sfix(16)  OutScaling=2^0
  ne : M-S-Function  Tag=ne  FunctionName=ltpdasim
  Out1 : Outport  OutDataType=sfix(16)  OutScaling=2^0
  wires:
  In1/1 -> ne/1
  ne/1 -> Out1/1

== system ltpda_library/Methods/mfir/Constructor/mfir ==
  Ground : Ground
  mfir : M-S-Function  Tag=mfir  FunctionName=ltpdasim
  Out1 : Outport  OutDataType=sfix(16)  OutScaling=2^0
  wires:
  Ground/1 -> mfir/1
  mfir/1 -> Out1/1

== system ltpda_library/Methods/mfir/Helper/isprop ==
  In1 : Inport  OutDataType=sfix(16)  OutScaling=2^0
  isprop : M-S-Function  Tag=isprop  FunctionName=ltpdasim
  Out1 : Outport  OutDataType=sfix(16)  OutScaling=2^0
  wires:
  In1/1 -> isprop/1
  isprop/1 -> Out1/1

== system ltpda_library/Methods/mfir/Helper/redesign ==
  In1 : Inport  OutDataType=sfix(16)  OutScaling=2^0
  redesign : M-S-Function  Tag=redesign  FunctionName=ltpdasim
  Out1 : Outport  OutDataType=sfix(16)  OutScaling=2^0
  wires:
  In1/1 -> redesign/1
  redesign/1 -> Out1/1

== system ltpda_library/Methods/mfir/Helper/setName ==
  In1 : Inport  OutDataType=sfix(16)  OutScaling=2^0
  setName : M-S-Function  Tag=setName  FunctionName=ltpdasim
  Out1 : Outport  OutDataType=sfix(16)  OutScaling=2^0
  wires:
  In1/1 -> setName/1
  setName/1 -> Out1/1

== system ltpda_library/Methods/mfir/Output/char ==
  In1 : Inport  OutDataType=sfix(16)  OutScaling=2^0
  Terminator : Terminator
  char : M-S-Function  Tag=char  FunctionName=ltpdasim
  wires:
  char/1 -> Terminator/1
  In1/1 -> char/1

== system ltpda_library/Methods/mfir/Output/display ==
  In1 : Inport  OutDataType=sfix(16)  OutScaling=2^0
  Terminator : Terminator
  display : M-S-Function  Tag=display  FunctionName=ltpdasim
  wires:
  display/1 -> Terminator/1
  In1/1 -> display/1

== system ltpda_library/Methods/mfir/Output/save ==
  In1 : Inport  OutDataType=sfix(16)  OutScaling=2^0
  Terminator : Terminator
  save : M-S-Function  Tag=save  FunctionName=ltpdasim
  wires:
  save/1 -> Terminator/1
  In1/1 -> save/1

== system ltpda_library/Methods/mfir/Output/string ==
  In1 : Inport  OutDataType=sfix(16)  OutScaling=2^0
  Terminator : Terminator
  string : M-S-Function  Tag=string  FunctionName=ltpdasim
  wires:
  string/1 -> Terminator/1
  In1/1 -> string/1

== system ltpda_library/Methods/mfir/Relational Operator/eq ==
  In1 : Inport  OutDataType=sfix(16)  OutScaling=2^0
  eq : M-S-Function  Tag=eq  FunctionName=ltpdasim
  Out1 : Outport  OutDataType=sfix(16)  OutScaling=2^0
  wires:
  In1/1 -> eq/1
  eq/1 -> Out1/1

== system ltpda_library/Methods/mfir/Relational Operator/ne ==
  In1 : Inport  OutDataType=sfix(16)  OutScaling=2^0
  ne : M-S-Function  Tag=ne  FunctionName=ltpdasim
  Out1 : Outport  OutDataType=sfix(16)  OutScaling=2^0
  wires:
  In1/1 -> ne/1
  ne/1 -> Out1/1

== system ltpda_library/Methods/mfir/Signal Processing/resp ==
  In1 : Inport  OutDataType=sfix(16)  OutScaling=2^0
  resp : M-S-Function  Tag=resp  FunctionName=ltpdasim
  Out1 : Outport  OutDataType=sfix(16)  OutScaling=2^0
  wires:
  In1/1 -> resp/1
  resp/1 -> Out1/1

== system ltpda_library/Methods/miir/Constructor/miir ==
  Ground : Ground
  miir : M-S-Function  Tag=miir  FunctionName=ltpdasim
  Out1 : Outport  OutDataType=sfix(16)  OutScaling=2^0
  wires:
  Ground/1 -> miir/1
  miir/1 -> Out1/1

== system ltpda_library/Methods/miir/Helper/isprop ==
  In1 : Inport  OutDataType=sfix(16)  OutScaling=2^0
  isprop : M-S-Function  Tag=isprop  FunctionName=ltpdasim
  Out1 : Outport  OutDataType=sfix(16)  OutScaling=2^0
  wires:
  In1/1 -> isprop/1
  isprop/1 -> Out1/1

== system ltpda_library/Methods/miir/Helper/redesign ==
  In1 : Inport  OutDataType=sfix(16)  OutScaling=2^0
  redesign : M-S-Function  Tag=redesign  FunctionName=ltpdasim
  Out1 : Outport  OutDataType=sfix(16)  OutScaling=2^0
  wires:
  In1/1 -> redesign/1
  redesign/1 -> Out1/1

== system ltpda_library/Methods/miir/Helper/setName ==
  In1 : Inport  OutDataType=sfix(16)  OutScaling=2^0
  setName : M-S-Function  Tag=setName  FunctionName=ltpdasim
  Out1 : Outport  OutDataType=sfix(16)  OutScaling=2^0
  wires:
  In1/1 -> setName/1
  setName/1 -> Out1/1

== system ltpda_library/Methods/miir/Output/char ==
  In1 : Inport  OutDataType=sfix(16)  OutScaling=2^0
  Terminator : Terminator
  char : M-S-Function  Tag=char  FunctionName=ltpdasim
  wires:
  char/1 -> Terminator/1
  In1/1 -> char/1

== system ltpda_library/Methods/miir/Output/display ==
  In1 : Inport  OutDataType=sfix(16)  OutScaling=2^0
  Terminator : Terminator
  display : M-S-Function  Tag=display  FunctionName=ltpdasim
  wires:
  display/1 -> Terminator/1
  In1/1 -> display/1

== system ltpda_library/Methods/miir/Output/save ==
  In1 : Inport  OutDataType=sfix(16)  OutScaling=2^0
  Terminator : Terminator
  save : M-S-Function  Tag=save  FunctionName=ltpdasim
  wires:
  save/1 -> Terminator/1
  In1/1 -> save/1

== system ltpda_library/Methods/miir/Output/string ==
  In1 : Inport  OutDataType=sfix(16)  OutScaling=2^0
  Terminator : Terminator
  string : M-S-Function  Tag=string  FunctionName=ltpdasim
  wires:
  string/1 -> Terminator/1
  In1/1 -> string/1

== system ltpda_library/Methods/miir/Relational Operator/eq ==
  In1 : Inport  OutDataType=sfix(16)  OutScaling=2^0
  eq : M-S-Function  Tag=eq  FunctionName=ltpdasim
  Out1 : Outport  OutDataType=sfix(16)  OutScaling=2^0
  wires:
  In1/1 -> eq/1
  eq/1 -> Out1/1

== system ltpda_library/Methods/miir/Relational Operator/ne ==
  In1 : Inport  OutDataType=sfix(16)  OutScaling=2^0
  ne : M-S-Function  Tag=ne  FunctionName=ltpdasim
  Out1 : Outport  OutDataType=sfix(16)  OutScaling=2^0
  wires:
  In1/1 -> ne/1
  ne/1 -> Out1/1

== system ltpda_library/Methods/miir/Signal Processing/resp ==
  In1 : Inport  OutDataType=sfix(16)  OutScaling=2^0
  resp : M-S-Function  Tag=resp  FunctionName=ltpdasim
  Out1 : Outport  OutDataType=sfix(16)  OutScaling=2^0
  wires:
  In1/1 -> resp/1
  resp/1 -> Out1/1

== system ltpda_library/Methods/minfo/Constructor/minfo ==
  Ground : Ground
  minfo : M-S-Function  Tag=minfo  FunctionName=ltpdasim
  Out1 : Outport  OutDataType=sfix(16)  OutScaling=2^0
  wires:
  Ground/1 -> minfo/1
  minfo/1 -> Out1/1

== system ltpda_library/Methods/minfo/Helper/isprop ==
  In1 : Inport  OutDataType=sfix(16)  OutScaling=2^0
  isprop : M-S-Function  Tag=isprop  FunctionName=ltpdasim
  Out1 : Outport  OutDataType=sfix(16)  OutScaling=2^0
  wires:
  In1/1 -> isprop/1
  isprop/1 -> Out1/1

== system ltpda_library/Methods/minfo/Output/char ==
  In1 : Inport  OutDataType=sfix(16)  OutScaling=2^0
  Terminator : Terminator
  char : M-S-Function  Tag=char  FunctionName=ltpdasim
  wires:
  char/1 -> Terminator/1
  In1/1 -> char/1

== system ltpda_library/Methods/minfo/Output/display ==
  In1 : Inport  OutDataType=sfix(16)  OutScaling=2^0
  Terminator : Terminator
  display : M-S-Function  Tag=display  FunctionName=ltpdasim
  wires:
  display/1 -> Terminator/1
  In1/1 -> display/1

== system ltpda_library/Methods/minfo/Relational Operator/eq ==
  In1 : Inport  OutDataType=sfix(16)  OutScaling=2^0
  eq : M-S-Function  Tag=eq  FunctionName=ltpdasim
  Out1 : Outport  OutDataType=sfix(16)  OutScaling=2^0
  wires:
  In1/1 -> eq/1
  eq/1 -> Out1/1

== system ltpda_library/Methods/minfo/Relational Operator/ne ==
  In1 : Inport  OutDataType=sfix(16)  OutScaling=2^0
  ne : M-S-Function  Tag=ne  FunctionName=ltpdasim
  Out1 : Outport  OutDataType=sfix(16)  OutScaling=2^0
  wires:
  In1/1 -> ne/1
  ne/1 -> Out1/1

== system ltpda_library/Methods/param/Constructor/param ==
  Ground : Ground
  param : M-S-Function  Tag=param  FunctionName=ltpdasim
  Out1 : Outport  OutDataType=sfix(16)  OutScaling=2^0
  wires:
  Ground/1 -> param/1
  param/1 -> Out1/1

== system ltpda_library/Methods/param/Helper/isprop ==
  In1 : Inport  OutDataType=sfix(16)  OutScaling=2^0
  isprop : M-S-Function  Tag=isprop  FunctionName=ltpdasim
  Out1 : Outport  OutDataType=sfix(16)  OutScaling=2^0
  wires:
  In1/1 -> isprop/1
  isprop/1 -> Out1/1

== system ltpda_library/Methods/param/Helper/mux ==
  In1 : Inport  OutDataType=sfix(16)  OutScaling=2^0
  mux : M-S-Function  Tag=mux  FunctionName=ltpdasim
  Out1 : Outport  OutDataType=sfix(16)  OutScaling=2^0
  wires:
  In1/1 -> mux/1
  mux/1 -> Out1/1

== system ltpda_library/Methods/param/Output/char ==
  In1 : Inport  OutDataType=sfix(16)  OutScaling=2^0
  Terminator : Terminator
  char : M-S-Function  Tag=char  FunctionName=ltpdasim
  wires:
  char/1 -> Terminator/1
  In1/1 -> char/1

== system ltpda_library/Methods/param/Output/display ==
  In1 : Inport  OutDataType=sfix(16)  OutScaling=2^0
  Terminator : Terminator
  display : M-S-Function  Tag=display  FunctionName=ltpdasim
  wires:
  display/1 -> Terminator/1
  In1/1 -> display/1

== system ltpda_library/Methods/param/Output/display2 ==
  In1 : Inport  OutDataType=sfix(16)  OutScaling=2^0
  Terminator : Terminator
  display2 : M-S-Function  Tag=display2  FunctionName=ltpdasim
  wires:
  display2/1 -> Terminator/1
  In1/1 -> display2/1

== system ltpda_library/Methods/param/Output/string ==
  In1 : Inport  OutDataType=sfix(16)  OutScaling=2^0
  Terminator : Terminator
  string : M-S-Function  Tag=string  FunctionName=ltpdasim
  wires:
  string/1 -> Terminator/1
  In1/1 -> string/1

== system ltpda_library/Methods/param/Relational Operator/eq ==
  In1 : Inport  OutDataType=sfix(16)  OutScaling=2^0
  eq : M-S-Function  Tag=eq  FunctionName=ltpdasim
  Out1 : Outport  OutDataType=sfix(16)  OutScaling=2^0
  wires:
  In1/1 -> eq/1
  eq/1 -> Out1/1

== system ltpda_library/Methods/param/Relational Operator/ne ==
  In1 : Inport  OutDataType=sfix(16)  OutScaling=2^0
  ne : M-S-Function  Tag=ne  FunctionName=ltpdasim
  Out1 : Outport  OutDataType=sfix(16)  OutScaling=2^0
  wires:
  In1/1 -> ne/1
  ne/1 -> Out1/1

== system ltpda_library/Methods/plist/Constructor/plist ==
  Ground : Ground
  plist : M-S-Function  Tag=plist  FunctionName=ltpdasim
  Out1 : Outport  OutDataType=sfix(16)  OutScaling=2^0
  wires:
  Ground/1 -> plist/1
  plist/1 -> Out1/1

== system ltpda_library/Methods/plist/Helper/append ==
  In1 : Inport  OutDataType=sfix(16)  OutScaling=2^0
  append : M-S-Function  Tag=append  FunctionName=ltpdasim
  Out1 : Outport  OutDataType=sfix(16)  OutScaling=2^0
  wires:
  In1/1 -> append/1
  append/1 -> Out1/1

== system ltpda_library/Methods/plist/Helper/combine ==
  In1 : Inport  OutDataType=sfix(16)  OutScaling=2^0
  combine : M-S-Function  Tag=combine  FunctionName=ltpdasim
  Out1 : Outport  OutDataType=sfix(16)  OutScaling=2^0
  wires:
  In1/1 -> combine/1
  combine/1 -> Out1/1

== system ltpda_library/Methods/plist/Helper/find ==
  In1 : Inport  OutDataType=sfix(16)  OutScaling=2^0
  find : M-S-Function  Tag=find  FunctionName=ltpdasim
  Out1 : Outport  OutDataType=sfix(16)  OutScaling=2^0
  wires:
  In1/1 -> find/1
  find/1 -> Out1/1

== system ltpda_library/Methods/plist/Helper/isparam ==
  In1 : Inport  OutDataType=sfix(16)  OutScaling=2^0
  isparam : M-S-Function  Tag=isparam  FunctionName=ltpdasim
  Out1 : Outport  OutDataType=sfix(16)  OutScaling=2^0
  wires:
  In1/1 -> isparam/1
  isparam/1 -> Out1/1

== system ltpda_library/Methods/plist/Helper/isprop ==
  In1 : Inport  OutDataType=sfix(16)  OutScaling=2^0
  isprop : M-S-Function  Tag=isprop  FunctionName=ltpdasim
  Out1 : Outport  OutDataType=sfix(16)  OutScaling=2^0
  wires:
  In1/1 -> isprop/1
  isprop/1 -> Out1/1

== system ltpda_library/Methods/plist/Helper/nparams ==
  In1 : Inport  OutDataType=sfix(16)  OutScaling=2^0
  nparams : M-S-Function  Tag=nparams  FunctionName=ltpdasim
  Out1 : Outport  OutDataType=sfix(16)  OutScaling=2^0
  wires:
  In1/1 -> nparams/1
  nparams/1 -> Out1/1

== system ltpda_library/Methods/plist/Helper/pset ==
  In1 : Inport  OutDataType=sfix(16)  OutScaling=2^0
  pset : M-S-Function  Tag=pset  FunctionName=ltpdasim
  Out1 : Outport  OutDataType=sfix(16)  OutScaling=2^0
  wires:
  In1/1 -> pset/1
  pset/1 -> Out1/1

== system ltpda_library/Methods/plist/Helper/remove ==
  In1 : Inport  OutDataType=sfix(16)  OutScaling=2^0
  remove : M-S-Function  Tag=remove  FunctionName=ltpdasim
  Out1 : Outport  OutDataType=sfix(16)  OutScaling=2^0
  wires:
  In1/1 -> remove/1
  remove/1 -> Out1/1

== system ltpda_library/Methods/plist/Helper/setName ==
  In1 : Inport  OutDataType=sfix(16)  OutScaling=2^0
  setName : M-S-Function  Tag=setName  FunctionName=ltpdasim
  Out1 : Outport  OutDataType=sfix(16)  OutScaling=2^0
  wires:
  In1/1 -> setName/1
  setName/1 -> Out1/1

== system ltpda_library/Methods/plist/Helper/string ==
  In1 : Inport  OutDataType=sfix(16)  OutScaling=2^0
  string : M-S-Function  Tag=string  FunctionName=ltpdasim
  Out1 : Outport  OutDataType=sfix(16)  OutScaling=2^0
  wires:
  In1/1 -> string/1
  string/1 -> Out1/1

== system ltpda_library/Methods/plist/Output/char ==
  In1 : Inport  OutDataType=sfix(16)  OutScaling=2^0
  Terminator : Terminator
  char : M-S-Function  Tag=char  FunctionName=ltpdasim
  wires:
  char/1 -> Terminator/1
  In1/1 -> char/1

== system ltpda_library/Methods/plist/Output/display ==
  In1 : Inport  OutDataType=sfix(16)  OutScaling=2^0
  Terminator : Terminator
  display : M-S-Function  Tag=display  FunctionName=ltpdasim
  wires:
  display/1 -> Terminator/1
  In1/1 -> display/1

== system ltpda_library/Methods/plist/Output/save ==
  In1 : Inport  OutDataType=sfix(16)  OutScaling=2^0
  Terminator : Terminator
  save : M-S-Function  Tag=save  FunctionName=ltpdasim
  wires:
  save/1 -> Terminator/1
  In1/1 -> save/1

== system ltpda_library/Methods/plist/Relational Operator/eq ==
  In1 : Inport  OutDataType=sfix(16)  OutScaling=2^0
  eq : M-S-Function  Tag=eq  FunctionName=ltpdasim
  Out1 : Outport  OutDataType=sfix(16)  OutScaling=2^0
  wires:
  In1/1 -> eq/1
  eq/1 -> Out1/1

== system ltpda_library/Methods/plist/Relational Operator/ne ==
  In1 : Inport  OutDataType=sfix(16)  OutScaling=2^0
  ne : M-S-Function  Tag=ne  FunctionName=ltpdasim
  Out1 : Outport  OutDataType=sfix(16)  OutScaling=2^0
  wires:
  In1/1 -> ne/1
  ne/1 -> Out1/1

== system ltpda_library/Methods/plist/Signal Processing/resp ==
  In1 : Inport  OutDataType=sfix(16)  OutScaling=2^0
  resp : M-S-Function  Tag=resp  FunctionName=ltpdasim
  Out1 : Outport  OutDataType=sfix(16)  OutScaling=2^0
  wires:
  In1/1 -> resp/1
  resp/1 -> Out1/1

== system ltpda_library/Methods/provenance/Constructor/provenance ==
  Ground : Ground
  provenance : M-S-Function  Tag=provenance  FunctionName=ltpdasim
  Out1 : Outport  OutDataType=sfix(16)  OutScaling=2^0
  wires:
  Ground/1 -> provenance/1
  provenance/1 -> Out1/1

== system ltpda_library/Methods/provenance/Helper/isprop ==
  In1 : Inport  OutDataType=sfix(16)  OutScaling=2^0
  isprop : M-S-Function  Tag=isprop  FunctionName=ltpdasim
  Out1 : Outport  OutDataType=sfix(16)  OutScaling=2^0
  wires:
  In1/1 -> isprop/1
  isprop/1 -> Out1/1

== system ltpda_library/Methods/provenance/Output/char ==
  In1 : Inport  OutDataType=sfix(16)  OutScaling=2^0
  Terminator : Terminator
  char : M-S-Function  Tag=char  FunctionName=ltpdasim
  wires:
  char/1 -> Terminator/1
  In1/1 -> char/1

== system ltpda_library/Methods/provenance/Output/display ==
  In1 : Inport  OutDataType=sfix(16)  OutScaling=2^0
  Terminator : Terminator
  display : M-S-Function  Tag=display  FunctionName=ltpdasim
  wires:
  display/1 -> Terminator/1
  In1/1 -> display/1

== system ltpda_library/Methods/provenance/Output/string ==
  In1 : Inport  OutDataType=sfix(16)  OutScaling=2^0
  Terminator : Terminator
  string : M-S-Function  Tag=string  FunctionName=ltpdasim
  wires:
  string/1 -> Terminator/1
  In1/1 -> string/1

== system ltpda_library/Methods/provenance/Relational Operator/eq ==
  In1 : Inport  OutDataType=sfix(16)  OutScaling=2^0
  eq : M-S-Function  Tag=eq  FunctionName=ltpdasim
  Out1 : Outport  OutDataType=sfix(16)  OutScaling=2^0
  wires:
  In1/1 -> eq/1
  eq/1 -> Out1/1

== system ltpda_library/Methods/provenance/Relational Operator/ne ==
  In1 : Inport  OutDataType=sfix(16)  OutScaling=2^0
  ne : M-S-Function  Tag=ne  FunctionName=ltpdasim
  Out1 : Outport  OutDataType=sfix(16)  OutScaling=2^0
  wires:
  In1/1 -> ne/1
  ne/1 -> Out1/1

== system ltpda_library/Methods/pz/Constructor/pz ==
  Ground : Ground
  pz : M-S-Function  Tag=pz  FunctionName=ltpdasim
  Out1 : Outport  OutDataType=sfix(16)  OutScaling=2^0
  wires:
  Ground/1 -> pz/1
  pz/1 -> Out1/1
